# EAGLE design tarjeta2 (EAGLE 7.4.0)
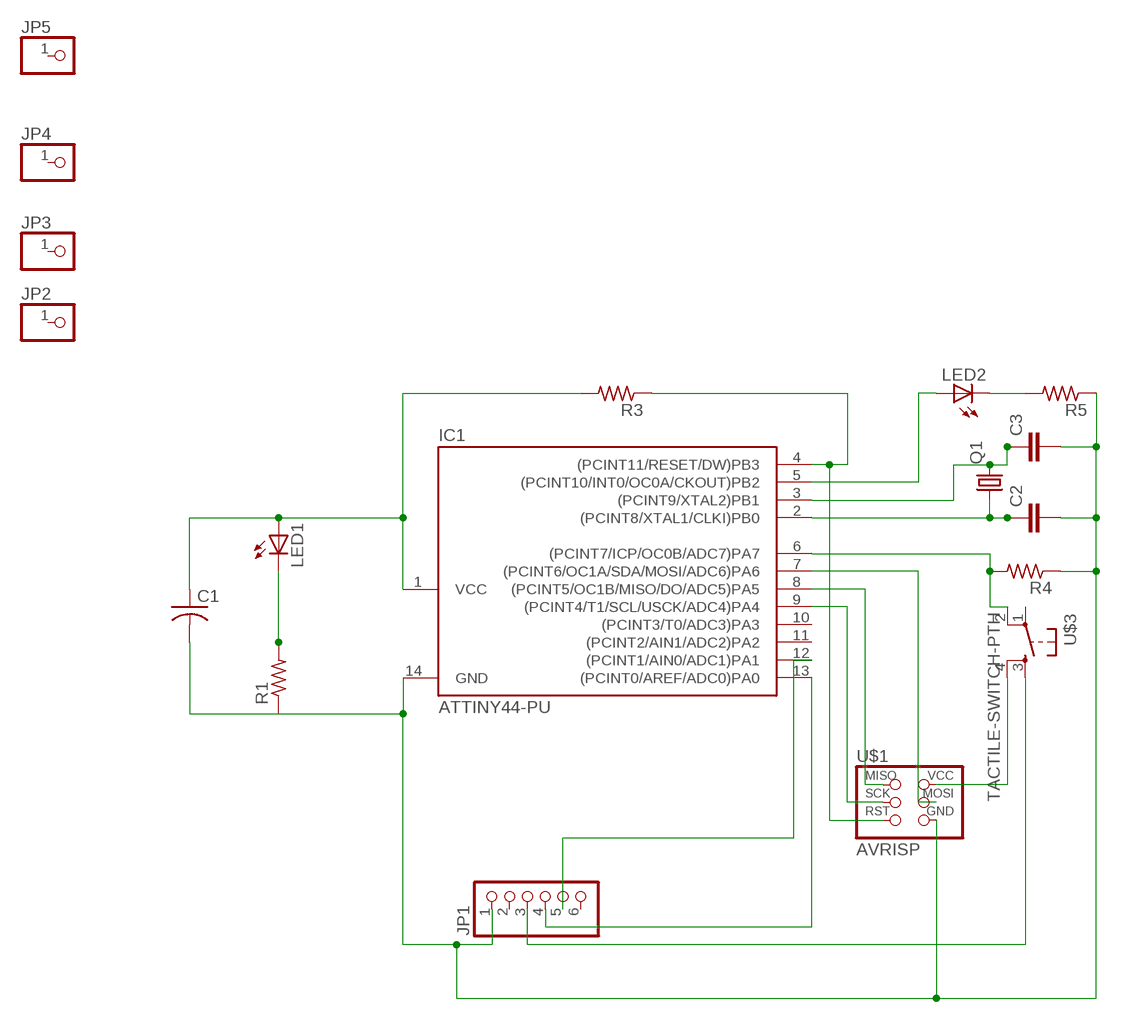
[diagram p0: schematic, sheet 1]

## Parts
C1  C-US025-024X044  [C025-024X044]
C2  C2,5-3  [C2.5-3]
C3  C2,5-3  [C2.5-3]
IC1  ATTINY44-PU  [DIL14]
JP1  PINHD-1X6  [1X06]
JP2  PINHD-1X1  [1X01]
JP3  PINHD-1X1  [1X01]
JP4  PINHD-1X1  [1X01]
JP5  PINHD-1X1  [1X01]
LED1  LED3MM  [LED3MM]
LED2  LED3MM  [LED3MM]
Q1  CRYSTALHC49S  [HC49/S]
R1  R-US_0204/5  [0204/5]
R3  R-US_0204/5  [0204/5]
R4  R-US_0204/5  [0204/5]
R5  R-US_0204/5  [0204/5]
U$1  AVRISP  [2X03]
U$3  TACTILE-SWITCH-PTH  [TAC-SWITCH-PTH]

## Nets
N$1: C1.1 IC1.1(VCC) LED1.A R3.2
N$2: LED1.K(C) R1.2
N$3: C1.2 C2.2 C3.2 IC1.14(GND) JP1.1 R1.1 R4.1 R5.1 U$1.6(GND)
N$4: IC1.4((PCINT11/RESET/DW)PB3) R3.1 U$1.5(RST)
N$5: IC1.9((PCINT4/T1/SCL/USCK/ADC4)PA4) U$1.3(SCK)
N$6: IC1.8((PCINT5/OC1B/MISO/DO/ADC5)PA5) U$1.1(MISO)
N$7: U$1.2(VCC) U$3.4
N$8: JP1.3 U$3.3
N$9: IC1.7((PCINT6/OC1A/SDA/MOSI/ADC6)PA6) U$1.4(MOSI)
N$10: IC1.6((PCINT7/ICP/OC0B/ADC7)PA7) R4.2 U$3.2
N$11: C2.1 IC1.2((PCINT8/XTAL1/CLKI)PB0) Q1.1
N$12: C3.1 IC1.3((PCINT9/XTAL2)PB1) Q1.2
N$13: IC1.5((PCINT10/INT0/OC0A/CKOUT)PB2) LED2.A
N$14: LED2.K(C) R5.2
N$15: IC1.13((PCINT0/AREF/ADC0)PA0) JP1.4
N$16: IC1.12((PCINT1/AIN0/ADC1)PA1) JP1.5
Unconnected: IC1.10((PCINT3/T0/ADC3)PA3) IC1.11((PCINT2/AIN1/ADC2)PA2) JP1.2 JP1.6 JP2.1 JP3.1 JP4.1 JP5.1 U$3.1

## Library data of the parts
C1 = resistor:C-US: CAPACITOR, American symbol
C2 C3 = capacitor-wima:C: CAPACITOR
IC1 = fab:ATTINY44
JP1 = pinhead:PINHD-1X6: PIN HEADER
JP2-JP5 = pinhead:PINHD-1X1: PIN HEADER
LED1 LED2 = led:LED: LED
Q1 = crystal:CRYSTAL: CRYSTAL; OC_FARNELL: 1667008; OC_NEWARK: unknown
R1 R3-R5 = resistor:R-US_: RESISTOR, American symbol
U$1 = fab:AVRISP
U$3 = GeekAmmo:TACTILE-SWITCH: Tactile Switch 4 Pins, SPST NO

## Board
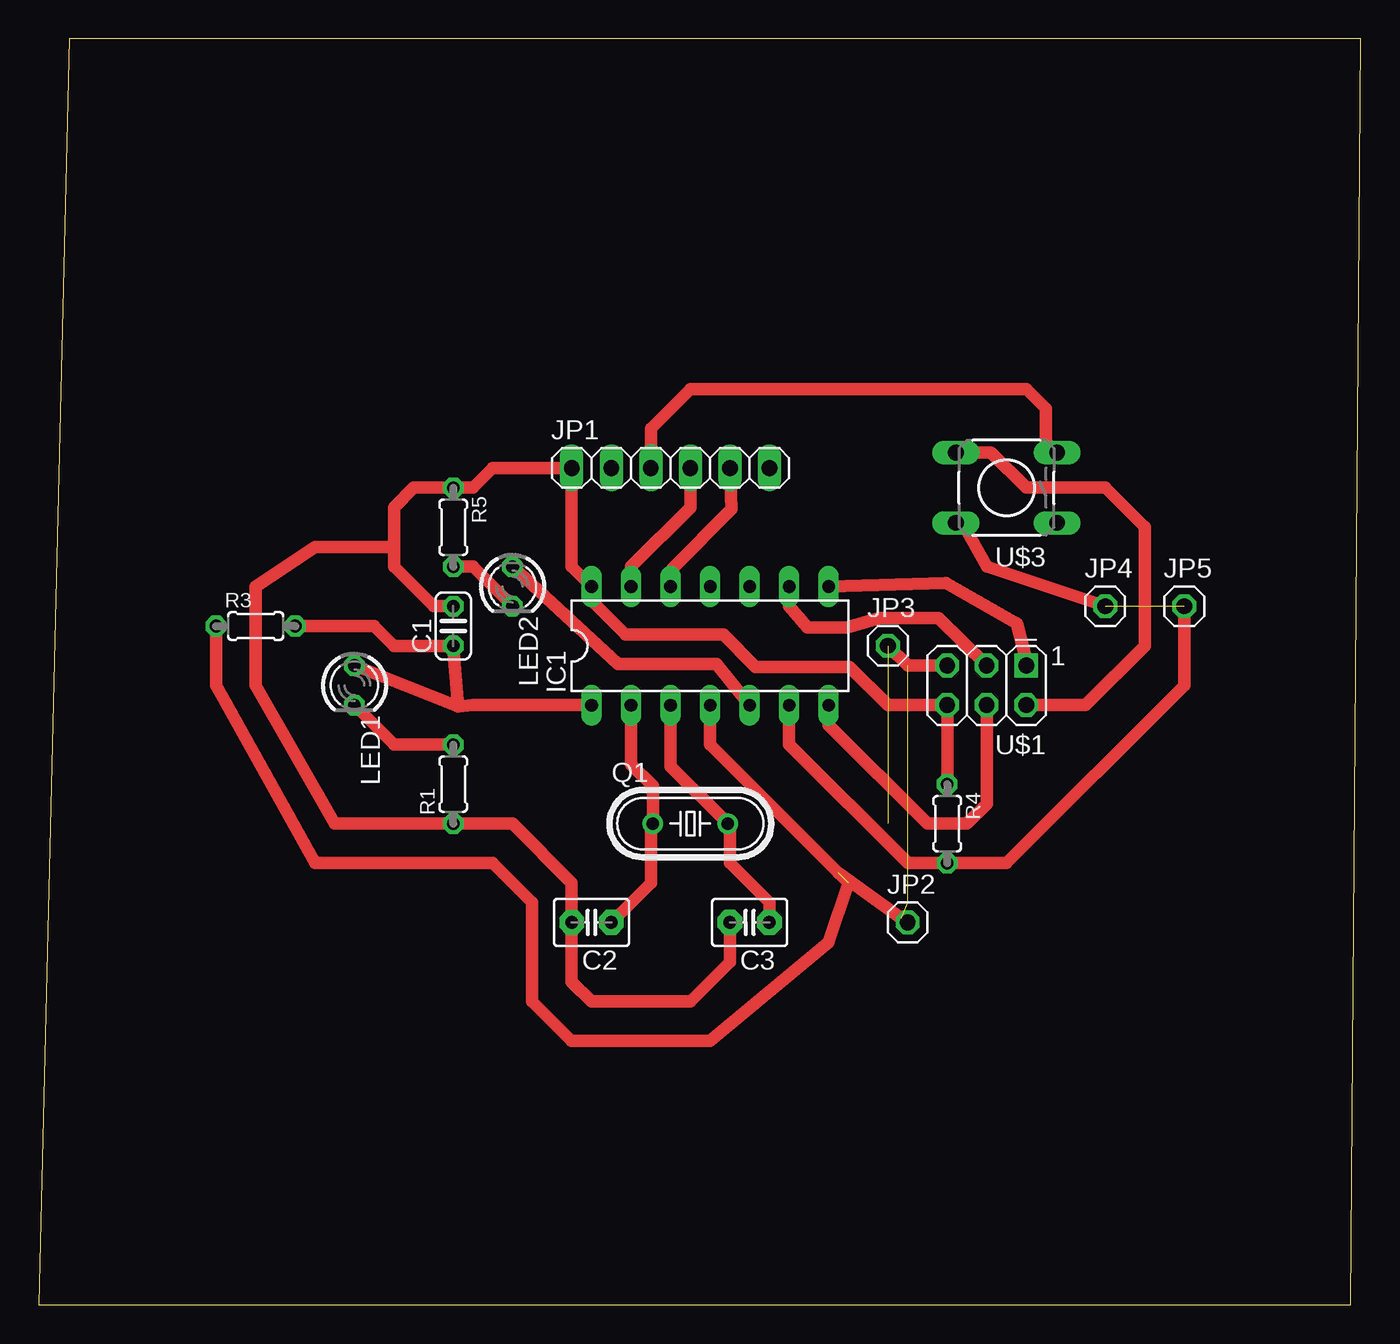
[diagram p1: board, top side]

Size 84.95 x 81.38 mm. Coordinates in mm from the lower left corner, seen from the top.
Outline: 0,0 84.31,0 84.95,81.38 1.96,81.38 0,0
Copper layers (1*16): Top 0.035mm / dielectric 1.5mm / Bottom 0.035mm
Design rules "default": minimum track width 10mil, minimum drill 24mil, track to track 8mil, track to pad 8mil, pad to pad 8mil, via to via 8mil, smd to smd 8mil, copper to edge 40mil, drill to drill 8mil, minimum pad ring 10mil, minimum via ring 8mil, stop-mask expansion 4mil, vias tented up to drill 0mil, thermal gap 10mil

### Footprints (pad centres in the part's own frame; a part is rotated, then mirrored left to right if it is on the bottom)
C025-024X044 = drill 0.813 octagon: 1 -1.27,0; 2 1.27,0
C2.5-3 = drill 0.813 pad 1.6 octagon: 1 -1.27,0; 2 1.27,0
DIL14 = drill 0.813 long: 1 -7.62,-3.81; 2 -5.08,-3.81; 3 -2.54,-3.81; 4 0,-3.81; 5 2.54,-3.81; 6 5.08,-3.81; 7 7.62,-3.81; 8 7.62,3.81; 9 5.08,3.81; 10 2.54,3.81; 11 0,3.81; 12 -2.54,3.81; 13 -5.08,3.81; 14 -7.62,3.81
1X06 = drill 1.016 long: 1 -6.35,0; 2 -3.81,0; 3 -1.27,0; 4 1.27,0; 5 3.81,0; 6 6.35,0
1X01 = drill 1.016 octagon: 1 0,0
LED3MM = drill 0.813 octagon: A -1.27,0; K 1.27,0
HC49/S = drill 0.813: 1 -2.413,0; 2 2.413,0
0204/5 = drill 0.813 octagon: 1 -2.54,0; 2 2.54,0
2X03 = drill 1.016 square: 1 -2.54,-1.27 | drill 1.016 octagon: 2 -2.54,1.27; 3 0,-1.27; 4 0,1.27; 5 2.54,-1.27; 6 2.54,1.27
TAC-SWITCH-PTH = drill 1.016 pad 1.524 long: 1 -3.251,2.261; 2 3.251,2.261; 3 -3.251,-2.261; 4 3.251,-2.261

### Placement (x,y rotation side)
C1  26.63,43.64 90 top
C2  35.52,24.59 180 top
C3  45.68,24.59 180 top
IC1  43.14,42.37 0 top
JP1  40.6,53.8 0 top
JP2  55.84,24.59 0 top
JP3  54.57,42.37 0 top
JP4  68.54,44.91 0 top
JP5  73.62,44.91 0 top
LED1  20.28,39.83 270 top
LED2  30.44,46.18 270 top
Q1  41.87,30.94 0 top
R1  26.63,33.48 90 top
R3  13.93,43.64 0 top
R4  58.38,30.94 270 top
R5  26.63,49.99 270 top
U$1  60.92,39.83 180 top
U$3  62.19,52.53 180 top

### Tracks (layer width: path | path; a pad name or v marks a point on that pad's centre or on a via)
N$1
  Top 0.813: 26.93,38.46 C1.1 22.82,42.37 21.55,43.64 R3.2 | LED1.A 26.93,38.46 | 26.93,38.46 27.9,38.56 IC1.1
N$2
  Top 0.813: LED1.K 22.82,36.02 R1.2
N$3
  Top 0.813: C3.2 44.41,22.05 41.87,19.51 35.52,19.51 34.25,20.78 C2.2 34.25,27.13 30.44,30.94 R1.1 19.01,30.94 13.93,39.83 13.93,46.18 17.74,48.72 22.82,48.72 | 22.82,48.72 22.82,51.26 24.09,52.53 R5.1 27.9,52.53 29.17,53.8 JP1.1 34.25,47.45 IC1.14 35.52,45.28 37.7,43.1 43.99,43.1 46.06,41.02 52.11,41.02 54.57,38.56 U$1.6 R4.1 | 22.82,48.72 22.82,47.45 25.36,44.91 C1.2
N$4  (4 unrouted)
  Top 0.813: R3.1 11.39,39.83 17.74,28.4 29.17,28.4 31.71,25.86 31.71,19.51 34.25,16.97 43.14,16.97 50.76,23.32 52.03,27.13 51.39,27.76 | 51.39,27.76 43.14,36.02 IC1.4 | U$1.5 55.84,41.1 54.57,42.37 | 51.39,27.76 55.45,24.85
N$5
  Top 0.813: IC1.9 48.22,44.91 49.39,43.53 51.93,43.53 54.01,44.15 57.82,44.15 U$1.3
N$6
  Top 0.813: IC1.8 58.3,46.41 62.85,43.79 63.54,41.17 U$1.1
N$7
  Top 0.813: U$3.4 61.2,54.79 63.46,52.53 68.54,52.53 71.08,49.99 71.08,42.37 67.27,38.56 U$1.2
N$8
  Top 0.813: JP1.3 39.33,56.34 41.87,58.88 63.46,58.88 64.73,57.61 64.73,55.5 U$3.3
N$9
  Top 0.813: IC1.7 50.76,37.29 57.11,30.94 59.65,30.94 60.92,32.21 U$1.4
N$10  (1 unrouted)
  Top 0.813: IC1.6 48.22,36.02 55.84,28.4 R4.2 62.19,28.4 73.62,39.83 73.62,44.91 | U$3.2 59.37,50.27 60.92,47.45 68.54,44.91
N$11
  Top 0.813: IC1.2 38.06,34.75 39.46,33.35 Q1.1 39.33,30.81 39.33,27.13 C2.1
N$12
  Top 0.813: C3.1 46.95,25.86 44.41,28.4 44.41,30.81 Q1.2 40.6,34.62 IC1.3
N$13
  Top 0.813: LED2.A 37.21,41.19 43.56,41.19 IC1.5
N$14
  Top 0.813: R5.2 27.9,47.45 LED2.K
N$15
  Top 0.813: IC1.13 38.06,47.45 41.87,51.26 JP1.4
N$16
  Top 0.813: IC1.12 40.72,47.33 44.53,51.14 JP1.5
